// TwinCAT 3 PLC project Local_Client
// ProgramVersion: 3.1.4020.4
// libraries:
//   Tc2_Standard, * (Beckhoff Automation GmbH)
//   Tc2_System, * (Beckhoff Automation GmbH)
//   Tc3_Module, * (Beckhoff Automation GmbH)
//   Tc3_PLCopen_OpcUa, * (Beckhoff Automation GmbH)
// project tree:
//   DUTs/ iState_Enum.TcDUT
//   / PlcTask.TcTTO
//   POUs/ Default_NN_Read.TcPOU, MAIN.TcPOU
// real-time tasks:
//   TASK PlcTask: cycle T#10ms, priority 20, ADS port 350

CONFIGURATION Local_Client
    RESOURCE PLC ON TwinCAT3
        TASK PlcTask(INTERVAL := T#10ms, PRIORITY := 20);
        PROGRAM MAIN WITH PlcTask : MAIN;
    END_RESOURCE
END_CONFIGURATION

// ---- DUTs/iState_Enum.TcDUT

TYPE iState_Enum :
(
	iState_Prepare			:= 0,
	iState_Connect			:= 1,
	iState_GetNameSpaceIndex:= 2,
	iState_GetNodeHandle	:= 3,
	iState_Read				:= 4,
	iState_ReleaseHandle	:= 5,
	iState_Disconnect		:= 6,
	iState_Error			:= 7
);
END_TYPE

// ---- POUs/MAIN.TcPOU
PROGRAM MAIN
VAR 
	i 			: INT;
	fbRead		: ARRAY[0..2] OF Default_NN_Read;
	nOut		: ARRAY[0..2] OF array[0..10 ] of INT;
	iState		: ARRAY[0..2] OF INT;
	bError		: ARRAY[0..2] OF BOOL;
	bBusy		: ARRAY[0..2] OF BOOL;
	nErrorID	: ARRAY[0..2] OF DWORD;
	Finish_Reading	: ARRAY[0..2] OF BOOL;
	
	ServerUrl	: STRING(MAX_STRING_LENGTH) := 'opc.tcp://192.168.0.2:4840';
	NameSpaceUri: STRING(MAX_STRING_LENGTH) := 'urn:CX-121E6A:BeckhoffAutomation:Ua:PLC1';
	NodeIdentifier	: ARRAY[0..2] OF STRING(MAX_STRING_LENGTH)	:= ['MAIN.structure_test.a', 'MAIN.iter2','MAIN.iteration3'];
END_VAR


	(*i := i + 1;
	IF i = 3 THEN
		i := 0;
	END_IF*)
	FOR i := 0 TO 2 BY 1 DO
		

	fbRead[i](
		ServerUrl_IN			:= ServerUrl,
		NameSpaceUri_IN			:= NameSpaceUri,
		NodeIdentifier_IN		:= NodeIdentifier[i],
		FinishReadingSignal_IN	:= Finish_Reading[i],
		iState_OUT				=> iState[i],
		Error_OUT				=> bError[i],
		Busy_OUT				=> bBusy[i],
		ErrorID_OUT				=> nErrorID[i],
		ReadingOntheNode_OUT	=> nOut[i]
	);
	END_FOR

END_PROGRAM

// ---- POUs/Default_NN_Read.TcPOU
FUNCTION_BLOCK Default_NN_Read
VAR_INPUT //输入
	ServerUrl_IN			:STRING(MAX_STRING_LENGTH); //IP地址
	NameSpaceUri_IN			:STRING(MAX_STRING_LENGTH); //PLC名称
	NodeIdentifier_IN		:STRING(MAX_STRING_LENGTH); //变量名称
	FinishReadingSignal_IN	:BOOL;						//结束读取信号
END_VAR
VAR_OUTPUT  //输出
	iState_OUT				:INT;						//输出当前状态
	Error_OUT				:BOOL;						//输出错误状态
	Busy_OUT				:BOOL;						//输出是否忙碌
	ErrorID_OUT				:DWORD;						//输出错误代码
	ReadingOntheNode_OUT	:ARRAY[0..10] OF INT;						//输出该变量读数
END_VAR 




VAR
	iState					:INT;
	bDone					:BOOL;
	bBusy					:BOOL;
	bError					:BOOL;
	nErrorID				:DWORD;
	
	//有一些基础的链接信息
	SessionConnectionInfo	:ST_UASessionConnectInfo;
	
	//获取连接句柄
	fbUA_Connect			:UA_Connect;
	nConnectionHdl			:DWORD;

	
	//获plc的句柄
	fbUA_GetNamespaceIndex	:UA_GetNamespaceIndex;
	nNamespaceIndex			:UINT;
	
	(*这一部分是用来获取变量句柄的程序及变量*)
	fbUA_NodeGetHandle		:UA_NodeGetHandle;
	stNodeID					:ST_UANodeID;
	nNodeHdl					:DWORD;
	
	
	
	(*这一部分是读取给定的变量的值，使用变量句柄*)
	fbUA_Read				:UA_Read;
	stNodeAddInfo			:ST_UANodeAdditionalInfo;
	nReadData				:INT;
	cbDataRead				:UDINT;
	
	(*这一部分是用来实现释放句柄与断开连接*)
	fbUA_NodeReleaseHandle	:UA_NodeReleaseHandle;
	fbUA_Disconnect			:UA_Disconnect;
END_VAR

//程序介绍: 这个功能块为Beckhoff 上海公司技术支持部门为帮助用户更好的理解程序而开发
//程序功能: 在设置正确的情况下持续读取一个IP地址中的一个带有OPCUA server 功能中的TwinCAT3控制器中的一个变量,
//			在只有一个本程序块运行的时候，读取周期为一个plc周期循环。在有终止信号进入的时候，将在三个plc周期内结束本程序
//程序作者: 鲁心源
//版本号:	version 1.0.2
//注意事项: 通过修改两行代码,本程序可在无加密 或 最高级加密之间进行切换,如果选用最高加密, 请详细阅读本程序附属文档

iState_Out					:= iState;		//本功能块是由 case 语句控制的有限状态机， iState 为 状态变量，默认值为0

CASE iState	OF
	
	//准备阶段
	iState_Prepare			:
		bDone				:= FALSE;
		bBusy				:= FALSE;
		bError				:= FALSE;
		nErrorID			:= 0;
		//SessionConnectionInfo 	 
		SessionConnectionInfo.tConnectTimeout		:= T#1M;		//定时器超时默认为一分钟
		SessionConnectionInfo.sApplicationName		:= '';
		//SessionConnectionInfo.eSecurityMode			:= eUASecurityMsgMode_Sign_Encrypt;		//数字签名且加密
		SessionConnectionInfo.eSecurityMode		:= eUASecurityMsgMode_None;				//不签名，不加密
		//SessionConnectionInfo.eSecurityPolicyUri	:= eUASecurityPolicy_Basic256;			//加密策略256
		SessionConnectionInfo.eSecurityPolicyUri	:= eUASecurityPolicy_None;				//无加密策略
		SessionConnectionInfo.eTransportProfileUri	:= eUATransportProfileUri_UATcp;			//UaTcp传输， 默认值为1
		iState 				:= iState_Connect;
		iState_OUT			:= iSTate;
	
	//连接阶段
	iState_Connect			:
		iState_OUT					:= iState;
		//Using library finction block here
		fbUA_Connect(
			Execute 				:= TRUE,
			ServerUrl				:= ServerUrl_IN,
			SessionConnectInfo		:= SessionConnectionInfo,
			Timeout					:= T#10S,
			ConnectionHdl 			=>nConnectionHdl, //连接句柄
			Busy					=>bBusy,
			Done					=>bDone,
			Error					=>bError,
			ErrorID					=>nErrorID
			);
		IF NOT bBusy	THEN
			fbUA_Connect(Execute	:= FALSE);
			IF NOT bError	THEN
				iState				:= iState_GetNameSpaceIndex;
			ELSE
				iState				:= iState_Prepare;
			END_IF
		END_IF
		
		
	//寻找命名空间索引阶段
	//本阶段我们将会获取要读取的PLC在命名空间中的索引
	//注意事项：我们不能直接从命名空间中将索引取出，因为索引数值可能会变，但命名空间的URI不会变，我们通过命名空间来获取索引值
	iState_GetNameSpaceIndex:
	fbUA_GetNamespaceIndex(
		Execute	:= TRUE,
		ConnectionHdl	:= nConnectionHdl, //之前获取到的连接句柄
		NamespaceUri	:= NameSpaceUri_IN,	//命名空间URI
		Timeout			:= T#5S,
		NamespaceIndex 	=> nNamespaceIndex,
		Done			=> bDone,
		Busy			=> bBusy,
		Error			=> bError,
		ErrorID			=> nErrorID
		);
		//判断是否出错
		IF NOT bBusy THEN
			fbUA_GetNamespaceIndex(Execute	:= FALSE);
			IF NOT bError THEN
				iState		:= iState_GetNodeHandle;
			ELSE
				iState		:= iState_Error;
			END_IF
		END_IF
	
	//获得节点句柄阶段
	//本小节用来获取节点句柄, 所谓节点, 就是变量
	iState_GetNodeHandle	:
		stNodeID.eIdentifierType	:= eUAIdentifierType_String; //变量识别符类型: 字符串
		stNodeID.nNamespaceIndex	:= nNamespaceIndex;			 //所在命名空间的索引，在上一个功能块中获得
		stNodeID.sIdentifier 		:= NodeIdentifier_IN;			//变量识别符本身, 即变量名
		fbUA_NodeGetHandle(
			Execute	:= TRUE,
			ConnectionHdl	:= nConnectionHdl,
			NodeID			:= stNodeID,
			Timeout			:= T#5S,
			NodeHdl			=> nNodeHdl,
			Done			=> bDone,
			Busy			=> bBusy,
			Error			=> bError,
			ErrorID			=> nErrorID
		);
		
		//判断出错的逻辑
		IF NOT bBusy THEN
			fbUA_NodeGetHandle(Execute:=FALSE);
			IF NOT bError THEN
				iState := iState + 1;
			END_IF
		END_IF
		
	//读取数值阶段
	iState_Read				:
		fbUA_Read(
			Execute		:= TRUE,
			ConnectionHdl	:= nConnectionHdl, //连接句柄
			NodeHdl			:= nNodeHdl, //变量句柄
			stNodeAddInfo	:= stNodeAddInfo, //一些附加信息，默认即可
			cbData 			:= SIZEOF(ReadingOntheNode_OUT),  //变量大小 
			pVariable		:= ADR(ReadingOntheNode_OUT),		//变量地址
			Timeout			:= T#5S,
			Done			=> bDone,
			Busy			=> bBusy,
			Error			=> bError,
			ErrorID			=> nErrorID,
			cbData_R		=> cbDataRead			//读到多少字节的信息
		);
		//错误判断
		IF NOT bBusy	THEN
			fbUA_Read(Execute := FALSE);
			IF NOT bError THEN
				//判断用户是否要结束读取
				IF NOT FinishReadingSignal_IN THEN 
					iState				:= iState; //利用plc周期达成循环
				ELSE
					iState				:= iState_ReleaseHandle;
				END_IF
			ELSE
				iState					:= iState;
			END_IF
		END_IF
		
	//释放句柄	
	iState_ReleaseHandle	:
		fbUA_NodeReleaseHandle(
			Execute			:= TRUE,
			ConnectionHdl	:= nConnectionHdl,
			NodeHdl			:= nNodeHdl,
			Timeout			:= DEFAULT_ADS_TIMEOUT,
			Done			=> bDone, 
			Busy			=> bBusy,
			Error			=> bError, 
			ErrorID			=> nErrorID
		);
		IF NOT bBusy	THEN
			fbUA_NodeReleaseHandle(Execute	:= FALSE);
			IF NOT bError THEN
				iState		:= iState_Disconnect;
			ELSE
				iState		:= iState_Error;
			END_IF
		END_IF
		
	//断开连接
	iState_Disconnect		:
		fbUA_Disconnect(
			Execute			:= TRUE,
			ConnectionHdl	:= nConnectionHdl,
			Timeout			:= DEFAULT_ADS_TIMEOUT, //ADS Timeout 
			Done			=> bDone,
			Busy			=> bBusy,
			Error			=> bError,
			ErrorID			=> nErrorID
		);
	iState_Error			:
		Error_OUT			:= bError;
		ErrorID_OUT			:= nErrorID;
END_CASE

END_FUNCTION_BLOCK
